FUNCTION_BLOCK FB_SampleA_Test
VAR_INPUT
	{attribute 'pytmc' := '
		pv: fInput
		io: io
	'}
	fInput : LREAL;
END_VAR
VAR_OUTPUT
	{attribute 'pytmc' := '
		pv: fOutput
		io: input
	'}
	fOutput : LREAL;
END_VAR
VAR
END_VAR

fOutput := fInput;

END_FUNCTION_BLOCK
